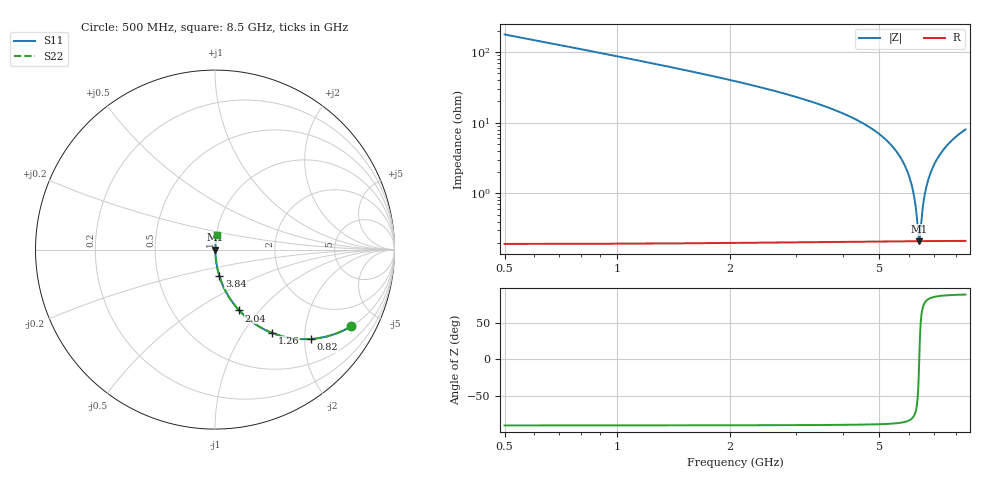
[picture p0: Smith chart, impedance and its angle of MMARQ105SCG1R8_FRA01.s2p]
! MMARQ105SCG1R8_FRA01  S-PARAMETER MODEL  ( General Type )
! Model Generated by TAIYO YUDEN Corporation (http://www.ty-top.com)
! Version 1.0
! TAIYO YUDEN Control No. 200326
! Copyright(c) 2020 TAIYO YUDEN CO.,LTD. All Rights Reserved.
! Product Description (link to TY-COMPAS)
! https://ds.yuden.co.jp/TYCOMPAS/or/detail?pn=MMARQ105SCG1R8BFRA01&u=M
! Products Name : Multilayer Ceramic Capacitors
! Characteristics :
!  Capacitance : 1.8 pF , Rated Voltage : 250V , TCC : CG / C0G
!  Case Size : 1.0 x 0.5 / 0.039 x 0.02 [mm/inch] , Thickness : 0.5 / 0.02 [mm/inch]
!  (Conditions: Temperature = 25 degC , DC Bias Current/Voltage = 0A / 0V)
! External Node Assignments :
!  1  o---| |---o  2
! GND o---------o GND
! Frequency Range : 500MHz  -  8.5GHz  [ 401 STEP ]
# MHz S RI R 50
! Freq[MHz].  S11 Real  S11 Imag  S21 Real  S21 Imag  S12 Real  S12 Imag  S22 Real  S22 Imag
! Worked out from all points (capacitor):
!   401 points, 500 MHz to 8.5 GHz, reference 50 ohm
!   read as one part in series: C = 1.78 pF near 540 MHz
!   lowest |Z| = 212 mohm at 6.4 GHz (marker M1)
!   series resonance near 6.4 GHz, so ESL is about 350 pH
!   S11 on the Smith chart (normalised r, x): 500 MHz: 1.00, -3.55; 820 MHz: 1.00, -2.14; 1.26 GHz: 1.00, -1.36; 2.04 GHz: 1.00, -0.79; 3.84 GHz: 1.00, -0.30; 8.5 GHz: 1.00, +0.16
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500  0.7586 -0.4274  0.2414 0.4274  0.2414 0.4274  0.7586 -0.4274
820  0.5339 -0.4979  0.4661 0.4979  0.4661 0.4979  0.5339 -0.4979
1260  0.3171 -0.4639  0.6829 0.4639  0.6829 0.4639  0.3171 -0.4639
1840  0.1663 -0.3701  0.8337 0.3701  0.8337 0.3701  0.1663 -0.3701
2040  0.135 -0.3392  0.865 0.3392  0.865 0.3392  0.135 -0.3392
3180  0.0445 -0.2015  0.9555 0.2015  0.9555 0.2015  0.0445 -0.2015
3840  0.0236 -0.1449  0.9764 0.1449  0.9764 0.1449  0.0236 -0.1449
4500  0.012 -0.0988  0.988 0.0988  0.988 0.0988  0.012 -0.0988
5300  0.00487 -0.0525  0.9951 0.0525  0.9951 0.0525  0.00487 -0.0525
5840  0.00275 -0.0254  0.9972 0.0254  0.9972 0.0254  0.00275 -0.0254
6020  0.0024 -0.017  0.9976 0.017  0.9976 0.017  0.0024 -0.017
6160  0.00222 -0.0106  0.9978 0.0106  0.9978 0.0106  0.00222 -0.0106
6240  0.00216 -0.00703  0.9978 0.00703  0.9978 0.00703  0.00216 -0.00703
6360  0.00211 -0.00175  0.9979 0.00175  0.9979 0.00175  0.00211 -0.00175
6400  0.00211 -7.84e-06  0.9979 7.84e-06  0.9979 7.84e-06  0.00211 -7.84e-06
6440  0.00211 0.00172  0.9979 -0.00172  0.9979 -0.00172  0.00211 0.00172
6560  0.00216 0.00685  0.9978 -0.00685  0.9978 -0.00685  0.00216 0.00685
6680  0.00226 0.0119  0.9977 -0.0119  0.9977 -0.0119  0.00226 0.0119
6880  0.00252 0.0201  0.9975 -0.0201  0.9975 -0.0201  0.00252 0.0201
7180  0.00314 0.0319  0.9969 -0.0319  0.9969 -0.0319  0.00314 0.0319
7740  0.00494 0.0529  0.9951 -0.0529  0.9951 -0.0529  0.00494 0.0529
8500  0.00847 0.0793  0.9915 -0.0793  0.9915 -0.0793  0.00847 0.0793
